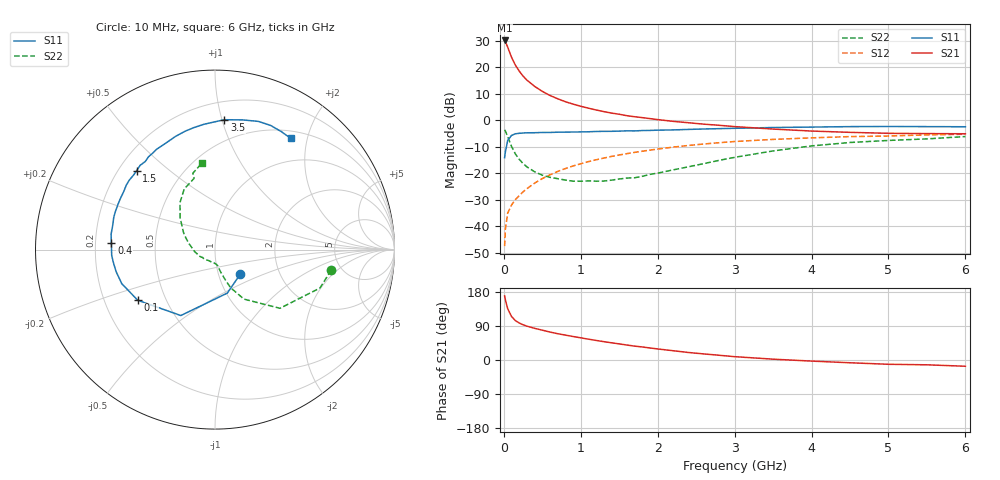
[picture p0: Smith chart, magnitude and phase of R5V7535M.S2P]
! SIEMENS Small Signal Semiconductors
! BFR183
! Si NPN RF Bipolar Junction Transistor in SOT23
! VCE = 0.75 V  IC = 35 mA
! Common Emitter S-Parameters:  May  1996
# GHz  S  MA  R  50
!  f  S11  S21  S12  S22
! GHz  MAG  ANG  MAG  ANG  MAG  ANG  MAG  ANG
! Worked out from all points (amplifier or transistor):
!   36 points, 10 MHz to 6 GHz, reference 50 ohm
!   highest |S21| = 30.0 dB at 10 MHz (marker M1)
!   |S21| within 3 dB of that: start of sweep to 56.24 MHz
!   unconditionally stable (mu >= 1): start of sweep to 25.2 MHz; 141.9 MHz to end of sweep
!   at 250 MHz: K = 1.18, MAG = 19.2 dB, |S12| = -27.0 dB
!   at 1.4 GHz: K = 1.25, MAG = 5.2 dB, |S12| = -13.7 dB
!   at 6 GHz: K = 1.07, MAG = -1.6 dB, |S12| = -5.3 dB
!   S11 on the Smith chart (normalised r, x): 10 MHz: 1.27, -0.36; 100 MHz: 0.35, -0.27; 400 MHz: 0.27, +0.03; 1.5 GHz: 0.27, +0.39; 3.5 GHz: 0.33, +1.02; 6 GHz: 0.61, +1.73
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0.01  0.1962 -44.2  31.77 169.1  0.0042 70.1  0.6575 -10.0
0.02  0.252 -74.2  30.32 158.6  0.0088 69.5  0.6229 -20.1
0.05  0.4137 -117.4  23.76 135.3  0.0176 62.4  0.4878 -42.1
0.1  0.5146 -146.7  15.31 114.8  0.0251 57.1  0.3194 -59.7
0.15  0.5529 -159.9  10.86 104.0  0.0317 59.8  0.2304 -67.6
0.2  0.5644 -167.4  8.401 97.6  0.0376 62.6  0.1825 -70.9
0.25  0.5714 -173.1  6.759 92.9  0.0445 64.5  0.1516 -73.3
0.3  0.5765 -176.9  5.675 89.3  0.0509 66.2  0.1313 -75.5
0.4  0.5786 176.2  4.329 83.6  0.0649 68.2  0.1063 -78.5
0.5  0.5851 171.6  3.485 78.7  0.079 68.6  0.0917 -80.5
0.6  0.5856 166.8  2.916 73.8  0.0931 68.5  0.0833 -84.0
0.7  0.592 162.3  2.525 69.4  0.1077 68.2  0.0787 -88.7
0.9  0.5963 155.0  2.003 62.0  0.1366 66.2  0.0705 -98.2
1.1  0.6025 147.6  1.679 55.0  0.1649 63.9  0.0715 -108.9
1.5  0.62 134.7  1.291 42.5  0.2201 58.1  0.0776 -134.2
1.7  0.6258 128.4  1.159 36.6  0.2464 55.1  0.0819 -148.3
2.2  0.6535 114.8  0.948 24.5  0.3098 46.9  0.1152 -175.1
3  0.701 95.0  0.755 8.8  0.3949 33.1  0.1987 151.8
3.5  0.7255 85.9  0.678 2.2  0.4331 24.9  0.2626 137.7
4.5  0.7541 71.3  0.588 -7.3  0.4889 10.6  0.3787 116.9
5.5  0.7541 60.6  0.557 -12.7  0.5275 -0.5  0.4429 106.2
6  0.7496 55.7  0.553 -16.5  0.5413 -7.5  0.4896 98.3
